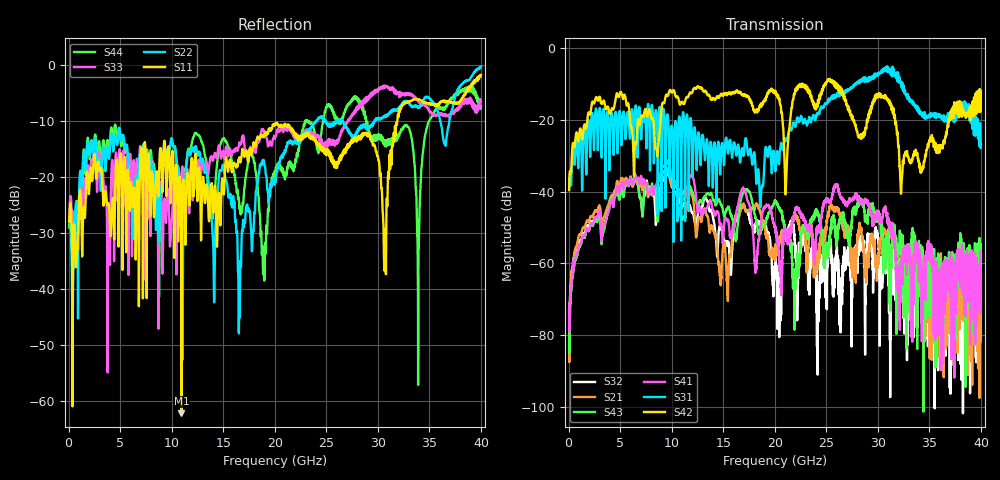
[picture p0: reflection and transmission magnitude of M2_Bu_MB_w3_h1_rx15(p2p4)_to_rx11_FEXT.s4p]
! S11 = S11
! S12 = S12
! S13 = S13
! S14 = S14
! S21 = S21
! S22 = S22
! S23 = S23
! S24 = S24
! S31 = S31
! S32 = S32
! S33 = S33
! S34 = S34
! S41 = S41
! S42 = S42
! S43 = S43
! S44 = S44
! FILE: \\englab.brocade.com\shares\Groups\SIT\Work\Shaohua\IEEE_channels\M2_Bu_MB_w3_h1_rx15(p2p4)_to_rx11_FEXT.s4p
!$DUT_CFG_DESC: Default 4-Port Configuration
!$NUMBER_PORTS: 4
!$DIFF_PORT_MAP: 1|2P|2|2P|0|UC|0|UC|
!$PORT_MAP: PNA 1|1|<<<<<<|TS 2|2|>>>>>>|PNA 2|3|<<<<<<|TS 4|4|>>>>>>|
# MHz S RI R 50.00
! FREQ  S11  S12  S13  S14
!  S21  S22  S23  S24
!  S31  S32  S33  S34
!  S41  S42  S43  S44
!  REAL  IMAG  REAL  IMAG  REAL  IMAG  REAL  IMAG
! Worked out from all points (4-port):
!   3996 points, 50 MHz to 40 GHz, reference 50 ohm
!   strongest paths, dB at 50 MHz, 10.04 GHz, 20.03 GHz, 30.02 GHz, 40 GHz:
!     S42: -39.5, -12.4, -12.3, -13.0, -11.9
!     S31: -39.6, -22.6, -33.5, -7.5, -26.9
!     S41: -72.7, -35.8, -49.5, -47.5, -64.8
!     S43: -74.7, -36.9, -42.9, -47.7, -56.9
!     S21: -73.1, -38.5, -57.3, -59.2, -80.2
!     S32: -83.6, -38.8, -61.5, -53.3, -71.8
!   lowest |S11| = -62.2 dB at 10.95 GHz (marker M1), VSWR 1.00, Z = 50.1 + j0.0431 ohm
!   |S11| at or under -10 dB: start of sweep to 31.89 GHz
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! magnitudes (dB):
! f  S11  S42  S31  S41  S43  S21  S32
! 50 MHz  -28.0  -39.5  -39.6  -72.7  -74.7  -73.1  -83.6
! 5.09 GHz  -16.6  -12.3  -23.6  -37.7  -39.9  -36.3  -38.9
! 10.95 GHz  -62.2  -15.0  -31.1  -42.2  -40.2  -47.7  -44.2
! 18.7 GHz  -12.8  -16.2  -39.7  -47.7  -50.5  -46.9  -48.8
! 30.65 GHz  -36.8  -13.3  -6.3  -45.0  -54.8  -50.8  -56.3
! 32.28 GHz  -7.7  -39.1  -10.2  -60.3  -53.9  -57.2  -69.5
! 40 GHz  -1.8  -11.9  -26.9  -64.8  -56.9  -80.2  -71.8
